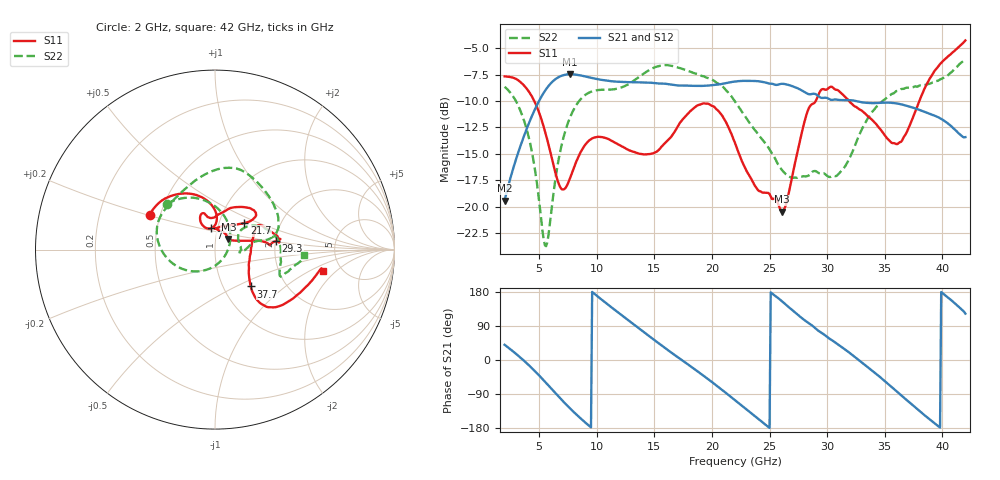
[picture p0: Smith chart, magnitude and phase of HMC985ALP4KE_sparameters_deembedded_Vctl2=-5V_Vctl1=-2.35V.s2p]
!s2p File: Measurements: S11, S21, S12, S22
# GHz S dB R 50.0
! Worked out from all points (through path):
!   401 points, 2 GHz to 42 GHz, reference 50 ohm
!   highest |S21| = -7.48 dB at 7.7 GHz (marker M1); lowest = -19.4 dB at 2 GHz (marker M2)
!   lowest |S11| = -20.4 dB at 26.1 GHz (marker M3), VSWR 1.21, Z = 57.6 + j6.85 ohm
!   |S11| at or under -10 dB: 4.573 GHz to 29.01 GHz (24.44 GHz wide, 146 % of centre); 31.9 GHz to 38 GHz (6.107 GHz wide, 17.5 % of centre)
!   |S22| runs from -23.7 to -6.1 dB; largest |S21 - S12| = 0.00055
!   S11 on the Smith chart (normalised r, x): 2 GHz: 0.44, +0.21; 7 GHz: 0.93, +0.22; 21.7 GHz: 1.32, +0.41; 29.3 GHz: 2.02, +0.21; 37.7 GHz: 1.34, -0.60; 42 GHz: 3.60, -1.34
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2  -7.68 151.9  -19.40 40.2  -19.40 40.2  -8.66 136.7
4  -8.95 118.7  -12.40 -10.8  -12.41 -10.8  -13.02 84.2
5.5  -12.84 91.2  -9.05 -57.1  -9.05 -57.1  -23.62 -21.7
7  -18.35 100.4  -7.60 -106.6  -7.60 -106.6  -13.92 -145.9
7.7  -17.23 114.8  -7.48 -128.4  -7.48 -128.3  -11.50 -168.1
8.7  -14.64 116.5  -7.61 -156.9  -7.61 -156.8  -9.72 169.2
10.3  -13.40 108.6  -7.99 162.3  -7.99 162.3  -8.95 145.8
12.3  -14.34 103.6  -8.21 115.1  -8.21 115.1  -8.66 121.0
15.4  -14.61 88.3  -8.35 43.6  -8.36 43.7  -6.70 80.4
18.3  -10.79 54.8  -8.57 -20.1  -8.57 -20.1  -7.31 50.9
20  -10.46 40.2  -8.51 -58.2  -8.51 -58.2  -7.98 28.7
21.7  -13.13 42.1  -8.21 -98.8  -8.21 -98.8  -9.58 12.4
22  -13.96 45.6  -8.16 -106.2  -8.17 -106.2  -10.04 11.3
24.1  -18.51 87.2  -8.15 -157.5  -8.15 -157.5  -13.29 10.7
26.1  -20.45 38.3  -8.38 154.4  -8.38 154.5  -16.55 -3.8
28.7  -10.29 4.6  -9.34 90.9  -9.34 91.0  -16.70 -1.0
29.3  -9.27 7.8  -9.60 75.8  -9.60 75.9  -16.82 2.0
32.4  -10.52 25.3  -9.99 8.1  -9.99 8.1  -14.26 37.0
35.4  -13.73 6.6  -10.16 -66.0  -10.16 -66.0  -9.52 15.4
37.7  -10.87 -45.9  -10.72 -126.4  -10.72 -126.3  -8.62 -6.2
39.7  -6.64 -43.5  -11.57 -176.0  -11.57 -175.9  -8.04 -22.3
42  -4.29 -11.0  -13.41 122.4  -13.41 122.4  -6.06 -3.4
